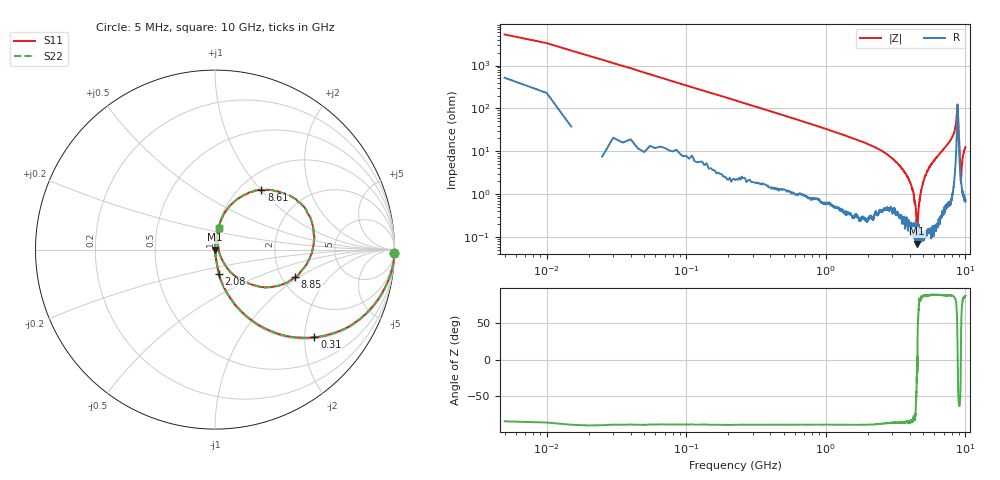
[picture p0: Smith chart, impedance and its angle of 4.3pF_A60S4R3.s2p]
! Amotech Co.,Ltd.
! http://www.amotech.co.kr/
! Part Number: A60S4R3
! These Parameters are Measured in Series Mode Connection
! Operation Temp=25[degC], DC Bias Voltage=0[V]
! Freq. Start=5[MHz] Stop=10[GHz], 2000[Steps]
! Date: Monday, July 13, 2020, 01:54:41
# GHZ S RI R 50.000000
!Freq.(Hz) S11(Real) S11(Imag) S21(Real) S21(Imag) S12(Real) S12(Imag) S22(Real) S22(Imag)
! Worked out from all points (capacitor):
!   2000 points, 5 MHz to 10 GHz, reference 50 ohm
!   read as one part in series: C = 4.64 pF near 55 MHz
!   lowest |Z| = 70.8 mohm at 4.52 GHz (marker M1)
!   series resonance near 4.514 GHz, so ESL is about 270 pH
!   S11 on the Smith chart (normalised r, x): 5 MHz: open; 310 MHz: 1.04, -2.23; 2.08 GHz: 1.01, -0.28; 8.61 GHz: 1.25, +1.01; 8.85 GHz: 2.36, -0.93; 10 GHz: 1.01, +0.25
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0.005  0.9978 -0.0188  0.00221 0.0188  0.00221 0.0188  0.9978 -0.0188
0.105  0.9094 -0.2769  0.0906 0.2769  0.0906 0.2769  0.9094 -0.2769
0.31  0.5535 -0.4887  0.4465 0.4887  0.4465 0.4887  0.5535 -0.4887
0.765  0.1692 -0.3655  0.8308 0.3655  0.8308 0.3655  0.1692 -0.3655
1.675  0.0364 -0.1786  0.9636 0.1786  0.9636 0.1786  0.0364 -0.1786
2.08  0.0223 -0.1369  0.9777 0.1369  0.9777 0.1369  0.0223 -0.1369
3.34  0.00547 -0.0473  0.9945 0.0473  0.9945 0.0473  0.00547 -0.0473
4.21  0.00164 -0.012  0.9984 0.012  0.9984 0.012  0.00164 -0.012
4.395  0.00157 -0.00494  0.9984 0.00494  0.9984 0.00494  0.00157 -0.00494
4.52  0.000697 -0.000124  0.9993 0.000124  0.9993 0.000124  0.000697 -0.000124
4.665  0.00136 0.006  0.9986 -0.006  0.9986 -0.006  0.00136 0.006
5.005  0.00128 0.02  0.9987 -0.02  0.9987 -0.02  0.00128 0.02
5.51  0.00325 0.0421  0.9968 -0.0421  0.9968 -0.0421  0.00325 0.0421
6.67  0.0119 0.0929  0.9881 -0.0929  0.9881 -0.0929  0.0119 0.0929
8.335  0.0924 0.2541  0.9076 -0.2541  0.9076 -0.2541  0.0924 0.2541
8.61  0.2585 0.3316  0.7415 -0.3316  0.7415 -0.3316  0.2585 0.3316
8.765  0.5421 0.1426  0.4579 -0.1426  0.4579 -0.1426  0.5421 0.1426
8.85  0.4466 -0.1536  0.5534 0.1536  0.5534 0.1536  0.4466 -0.1536
9.015  0.1068 -0.1437  0.8932 0.1437  0.8932 0.1437  0.1068 -0.1437
9.285  0.0196 0.00335  0.9804 -0.00335  0.9804 -0.00335  0.0196 0.00335
9.59  0.0158 0.0721  0.9842 -0.0721  0.9842 -0.0721  0.0158 0.0721
10  0.022 0.1223  0.978 -0.1223  0.978 -0.1223  0.022 0.1223
